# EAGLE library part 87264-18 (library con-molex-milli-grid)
RECEPTACAL
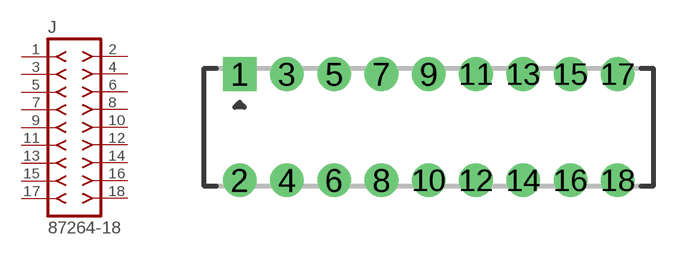
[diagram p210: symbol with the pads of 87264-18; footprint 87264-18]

Designator prefix J

## 87264-18  [87264-18]
1  1  pas
2  2  pas
3  3  pas
4  4  pas
5  5  pas
6  6  pas
7  7  pas
8  8  pas
9  9  pas
10  10  pas
11  11  pas
12  12  pas
13  13  pas
14  14  pas
15  15  pas
16  16  pas
17  17  pas
18  18  pas

## Footprint 87264-18 (pad centres in mm)
RECEPTACAL Dual Row, Side Entry
drill 0.914 square: 1 -8,2.25
drill 0.914: 2 -8,-2.25; 3 -6,2.25; 4 -6,-2.25; 5 -4,2.25; 6 -4,-2.25; 7 -2,2.25; 8 -2,-2.25; 9 0,2.25; 10 0,-2.25; 11 2,2.25; 12 2,-2.25; 13 4,2.25; 14 4,-2.25; 15 6,2.25; 16 6,-2.25; 17 8,2.25; 18 8,-2.25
